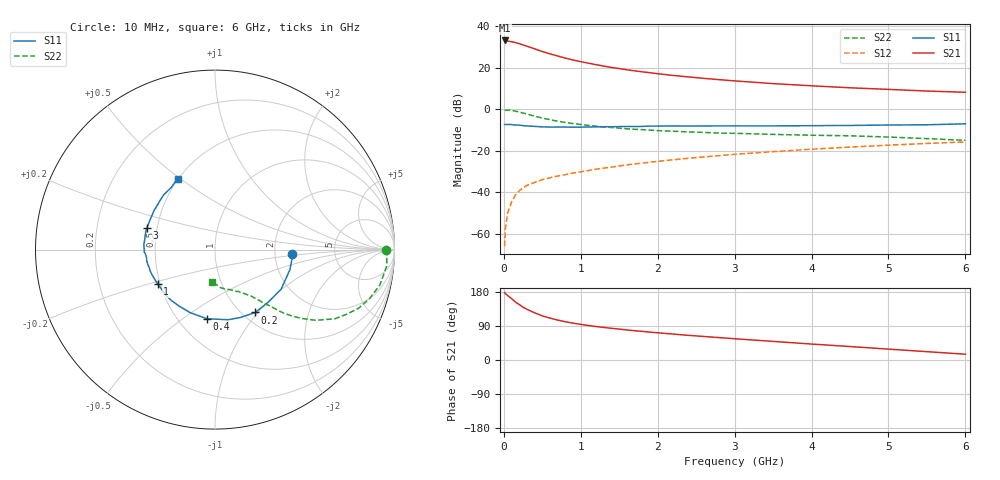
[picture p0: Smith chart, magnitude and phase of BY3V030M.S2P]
! SIEMENS Small Signal Semiconductors
! BFY420
! Si NPN RF SIEGET Grounded Emitter Transistor in MICRO-X
! VCE = 3 V  IC = 30 mA
! Common Emitter S-Parameters:  October  1996
# GHz  S  MA  R  50
!  f  S11  S21  S12  S22
! GHz  MAG  ANG  MAG  ANG  MAG  ANG  MAG  ANG
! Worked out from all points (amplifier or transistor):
!   36 points, 10 MHz to 6 GHz, reference 50 ohm
!   highest |S21| = 33.2 dB at 10 MHz (marker M1)
!   |S21| within 3 dB of that: start of sweep to 318.8 MHz
!   unconditionally stable (mu >= 1): start of sweep to 13.01 MHz; 1.66 GHz to end of sweep
!   at 250 MHz: K = 0.36, MSG = 34.5 dB, |S12| = -37.9 dB
!   at 1.4 GHz: K = 0.97, MSG = 24.0 dB, |S12| = -27.9 dB
!   at 6 GHz: K = 1.06, MAG = 10.5 dB, |S12| = -15.7 dB
!   S11 on the Smith chart (normalised r, x): 10 MHz: 2.51, -0.15; 200 MHz: 1.14, -0.97; 400 MHz: 0.68, -0.62; 1 GHz: 0.48, -0.21; 3 GHz: 0.44, +0.12; 6 GHz: 0.49, +0.49
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0.01  0.4312 -3.3  45.84 178.1  0.0005 118.3  0.9505 -0.1
0.02  0.4326 -5.9  45.56 175.2  0.0013 98.8  0.9578 -1.5
0.1  0.4294 -30.8  42.87 162.0  0.0058 78.6  0.9399 -12.0
0.15  0.4172 -44.3  40.68 153.1  0.0085 74.6  0.9039 -17.6
0.2  0.4158 -57.4  38.49 146.4  0.0108 72.2  0.8625 -22.4
0.25  0.4038 -69.6  35.85 139.4  0.0128 68.0  0.8127 -26.5
0.3  0.3974 -79.5  33.37 133.7  0.0146 66.8  0.7697 -30.1
0.4  0.3878 -96.8  28.8 124.6  0.0173 63.3  0.685 -35.1
0.5  0.3776 -111.4  24.8 116.4  0.0201 63.1  0.616 -38.5
0.6  0.3731 -122.1  21.8 110.6  0.0224 62.3  0.5614 -41.0
0.7  0.3734 -130.2  19.34 105.3  0.0245 62.4  0.5182 -42.9
0.8  0.3738 -137.6  17.19 101.0  0.0266 62.1  0.4815 -44.2
1  0.3724 -149.2  14.12 94.0  0.0311 62.2  0.4302 -46.1
1.1  0.3746 -153.9  12.97 91.1  0.0334 62.5  0.4097 -47.4
1.3  0.3801 -161.8  11.02 85.9  0.0382 62.4  0.3767 -48.8
1.6  0.3856 -170.6  8.992 79.2  0.0456 62.5  0.3394 -51.3
2.2  0.3974 176.0  6.567 68.4  0.0607 60.6  0.2968 -56.1
3  0.3986 162.7  4.852 56.1  0.0821 56.0  0.2638 -62.2
3.5  0.3981 154.3  4.172 49.1  0.0953 52.6  0.2486 -66.2
4.5  0.4083 140.1  3.307 35.5  0.1227 44.4  0.2297 -74.8
5.5  0.424 124.9  2.762 22.0  0.1505 35.1  0.1965 -87.5
6  0.4471 117.8  2.58 15.3  0.1633 30.3  0.1789 -96.1
